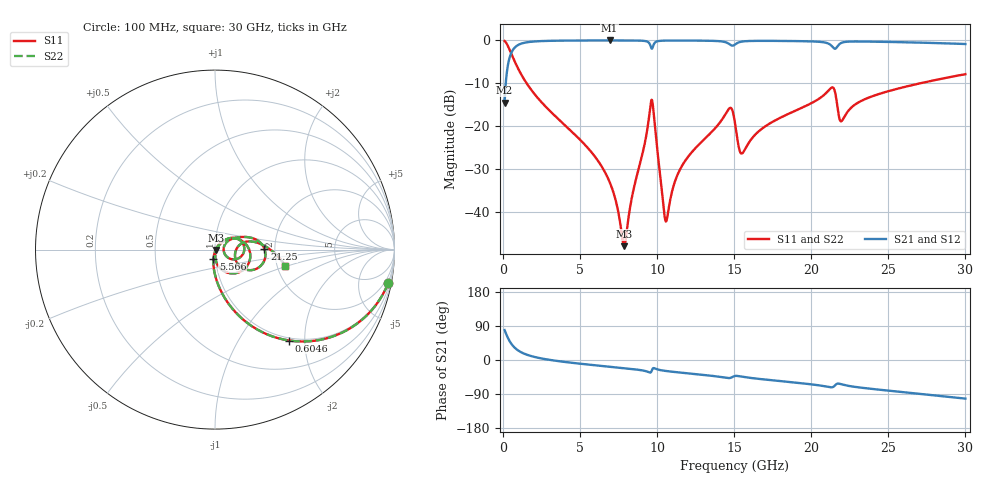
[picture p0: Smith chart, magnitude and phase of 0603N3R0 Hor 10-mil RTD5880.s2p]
# GHz S MA R 50
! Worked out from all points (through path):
!   3201 points, 100 MHz to 30 GHz, reference 50 ohm
!   highest |S21| = -0.03 dB at 6.912 GHz (marker M1); lowest = -14.6 dB at 100 MHz (marker M2)
!   group delay of S21, straight-line fit = 10.9 ps
!   lowest |S11| = -48.0 dB at 7.855 GHz (marker M3), VSWR 1.01, Z = 50.4 - j0.163 ohm
!   |S11| at or under -10 dB: 1.527 GHz to 27.08 GHz (25.55 GHz wide, 179 % of centre)
!   |S22| runs from -48.0 to -0.2 dB; largest |S21 - S12| = 0
!   S11 on the Smith chart (normalised r, x): 100 MHz: 1, -10; 604.6 MHz: 0.95, -1.69; 5.566 GHz: 0.98, -0.10; 21.25 GHz: 1.76, +0.01; 30 GHz: 2.22, -0.49
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0.1  0.9823 -11.1  0.1871 78.9  0.1871 78.9  0.9823 -11.1
0.6045625  0.6537 -50.8  0.756 39.2  0.756 39.2  0.6537 -50.8
1.725812  0.2807 -78.2  0.9583 11.5  0.9583 11.5  0.2807 -78.2
5.089563  0.06686 -97.9  0.995 -10.2  0.995 -10.2  0.06686 -97.9
5.566094  0.05402 -99.3  0.9957 -12.2  0.9957 -12.2  0.05402 -99.3
6.911594  0.02243 -99.2  0.9963 -17.7  0.9963 -17.7  0.02243 -99.2
7.855313  0.004001 -23.8  0.9959 -21.6  0.9959 -21.6  0.004001 -23.8
9.59325  0.1894 1.0  0.8361 -32.2  0.8361 -32.2  0.1894 1.0
9.752094  0.1542 -58.5  0.8726 -21.4  0.8726 -21.4  0.1542 -58.5
10.06978  0.04219 -88.0  0.9797 -25.4  0.9797 -25.4  0.04219 -88.0
10.59303  0.007843 -12.1  0.9924 -29.1  0.9924 -29.1  0.007843 -12.1
11.19103  0.02372 44.1  0.9938 -31.9  0.9938 -31.9  0.02372 44.1
11.94787  0.04263 47.5  0.9934 -35.0  0.9934 -35.0  0.04263 47.5
14.66691  0.1601 11.2  0.9077 -47.7  0.9077 -47.7  0.1601 11.2
15.05  0.1087 -29.7  0.8934 -42.1  0.8934 -42.1  0.1087 -29.7
15.51719  0.04822 5.1  0.9676 -44.1  0.9676 -44.1  0.04822 5.1
16.91875  0.09692 33.3  0.9858 -51.2  0.9858 -51.2  0.09692 33.3
20.03956  0.1867 22.1  0.9709 -64.4  0.9709 -64.4  0.1867 22.1
21.25425  0.2756 0.8  0.8829 -72.0  0.8829 -72.0  0.2756 0.8
21.96438  0.1146 -5.4  0.9354 -64.2  0.9354 -64.2  0.1146 -5.4
25.01978  0.256 7.1  0.9576 -80.9  0.9576 -80.9  0.256 7.1
30  0.4034 -13.2  0.9057 -101.9  0.9057 -101.9  0.4034 -13.2
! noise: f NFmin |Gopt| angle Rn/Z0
0.1  0.000397  0.9409  0.8508  0.0015
3.417  0.003988  0.8079  9.605  0.00429
6.743  0.006908  0.7848  18.6  0.006427
10.06  0.02101  0.889  27.56  0.03884
13.39  0.01572  0.8124  36.33  0.01581
16.7  0.01895  0.8083  45  0.0176
20.03  0.02202  0.8049  53.4  0.01877
23.35  0.02378  0.7932  61.66  0.01759
26.67  0.02228  0.7563  69.41  0.01261
30  0.02457  0.755  77.09  0.01254
